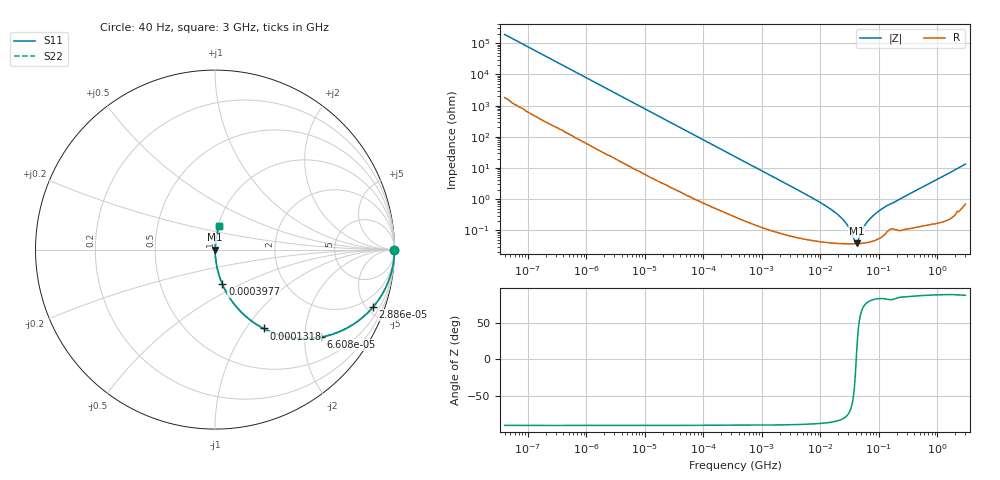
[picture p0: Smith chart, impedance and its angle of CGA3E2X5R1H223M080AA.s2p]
! S-parameter Generated by TDK Corporation
! Copyright(C) 2015 TDK Corporation.
! All Rights Reserved.
! TDK P/N: CGA3E2X5R1H223M080AA (Multilayer Ceramic Chip Capacitors)
! Property: C=22nF
! Size(LxWxT): 1.6x0.8x0.8mm, 0.063x0.031x0.031inches
! Model Type: s2p (Touchstone File Format Version 1.0)
! Frequency: DC=Yes Start=0.00004MHz Stop=3000MHz 396points Log-sweep
! Note: This model was converted from impedance.
! Model Generated on Jun. 23, 2015
! Hash(MD5):
! Port Assignments:
!  1 ---| |--- 2
! Applicable Conditions:
!  Temperature = 25 degC
!  DC Bias Voltage = 0 V
!  Small Signal Operation
! Terms and conditions regarding TDK Simulation Models
! (1)This simulation model is being provided solely for informational purposes. Please refer to the specifications of the products in terms of detailed characteristics of such products.
! (2)In no event shall TDK Corporation of any of its subsidiaries be liable for any loss or damage arising, directly or indirectly,
!  From any information contained in this simulation model, including, but not limited to loss or damages arising from any inaccuracies, omissions or errors in connection with such information.
! (3)Any and all copyrights on this simulation model are owned by TDK Corporation.
!  Duplication or redistribution of this simulation model without prior written permission from TDK Corporation is prohibited.
! (4)This simulation model is subject to any modification or change without any prior notice.
! (5)Neither TDK Corporation nor any of its subsidiaries shall make any warranty, express or implied,
!  Including but not limited to the correctness, implied warranties of merchantability and fitness for a particular purpose with respect to this simulation models.
! (6)The use of this simulation model shall be deemed to have consented to the terms and conditions hereof.
# MHz S MA R 50
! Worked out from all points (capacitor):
!   395 points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, 40 Hz to 3 GHz, reference 50 ohm
!   read as one part in series: C = 20.9 nF near 41.88 Hz
!   lowest |Z| = 38.3 mohm at 41.52 MHz (marker M1)
!   series resonance near 40.87 MHz, so ESL is about 730 pH
!   S11 on the Smith chart (normalised r, x): 40 Hz: open; 28.86 kHz: 1.05, -5.48; 66.08 kHz: 1.02, -2.41; 131.8 kHz: 1.01, -1.21; 397.7 kHz: 1.00, -0.40; 3 GHz: 1.01, +0.27
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4e-05  1 -0.0  0.0005249 89.4  0.0005249 89.4  1 -0.0
0.000834128  0.9999 -0.6  0.01073 88.9  0.01073 88.9  0.9999 -0.6
0.005256919  0.9972 -3.8  0.0668 85.7  0.0668 85.7  0.9972 -3.8
0.01739424  0.9749 -12.4  0.2149 77.1  0.2149 77.1  0.9749 -12.4
0.02885808  0.937 -20.0  0.3417 69.5  0.3417 69.5  0.937 -20.0
0.06607572  0.7656 -39.5  0.6366 50.0  0.6366 50.0  0.7656 -39.5
0.1317813  0.5158 -58.4  0.8517 31.0  0.8517 31.0  0.5158 -58.4
0.3464102  0.2254 -76.3  0.9717 13.0  0.9717 13.0  0.2254 -76.3
0.3976976  0.1978 -77.9  0.9779 11.4  0.9779 11.4  0.1978 -77.9
1.256723  0.06436 -85.4  0.9969 3.7  0.9969 3.7  0.06436 -85.4
7.22376  0.01106 -86.9  0.9995 0.6  0.9995 0.6  0.01106 -86.9
15.08561  0.004762 -85.0  0.9996 0.3  0.9996 0.3  0.004762 -85.0
22.82706  0.002533 -81.3  0.9996 0.1  0.9996 0.1  0.002533 -81.3
30.08671  0.00132 -73.7  0.9996 0.1  0.9996 0.1  0.00132 -73.7
39.65514  0.0003939 -18.2  0.9996 0.0  0.9996 0.0  0.0003939 -18.2
41.52283  0.0003827 9.9  0.9996 -0.0  0.9996 -0.0  0.0003827 9.9
52.26661  0.001086 68.9  0.9996 -0.1  0.9996 -0.1  0.001086 68.9
65.79027  0.002063 78.4  0.9996 -0.1  0.9996 -0.1  0.002063 78.4
90.7975  0.003669 81.9  0.9995 -0.2  0.9995 -0.2  0.003669 81.9
150.6385  0.006807 80.9  0.9989 -0.4  0.9989 -0.4  0.006807 80.9
949.3681  0.04161 85.3  0.9975 -2.4  0.9975 -2.4  0.04161 85.3
3000  0.1323 79.4  0.9844 -7.6  0.9844 -7.6  0.1323 79.4
